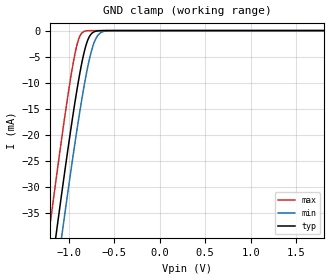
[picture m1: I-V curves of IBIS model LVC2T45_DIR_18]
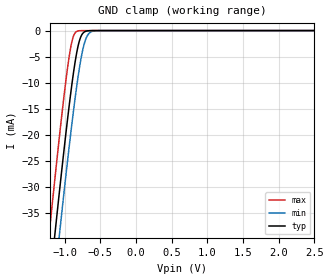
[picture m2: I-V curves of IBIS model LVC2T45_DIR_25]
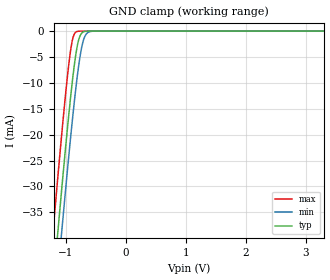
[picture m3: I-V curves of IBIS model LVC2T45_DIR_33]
| TEXAS INSTRUMENTS INCORPORATED
| Standard Linear and Logic Group
| IBIS Model of SN74LVC2T45
| 2-Bit Dual Supply Transceiver with Configurable Output Voltage
| This file contains package information for the following:
|  DSBGA 8-pin (YEP) package as [Component] LVC2T45_YEP
|  DSBGA 8-pin (YZP) package as [Component] LVC2T45_YZP
|  SOT 8-pin (DCT) package as [Component] LVC2T45_DCT
|  SOT 8-pin (DCU) package as [Component] LVC2T45_DCU
| This device can be powered at the following Vccs:
|  1.8 volt Vcc
|  2.5 volt Vcc
|  3.3 volt Vcc
|  5 volt Vcc
| This file provides unique models under the [Model Selector] for each Vcc.
| For operation at a specific Vcc, select the appropriate model after each
| [Model Selector] keyword.
[IBIS Ver]   3.2
[Comment char]  |_char
[File Name]   sn74lvc2t45.ibs
[File Rev]   1.2 | x_die
[Date]   April 30, 2004
[Source]   Data created from TI-SPICE simulations at TI-SLL.
[Notes]   The following is an IBIS list for the LVC2T45.
   Please contact sllibis@ti.com with questions and
   comments concerning SLL IBIS models.
   - FILE REV HISTORY
   - 1.1 Release IBIS file on 02/05/04
   - 1.2 YEP and YZP packages released 04/30/04
   - Due to the fact that the Device is 5-V Input/Output
   tolarent, the output model has some Non-Monotonic Warnings.
   - Power clamp data deleted as there is no power-clamp diode.
[Disclaimer] Property of Texas Instruments Incorporated.  Unauthorized
   reproduction and/or distribution is strictly prohibited.
   This product is protected under copyright law.
   Created  2003, (C) Copyright  2003, Texas Instruments
   Incorporated, All Rights Reserved
   UNLESS THERE IS A SIGNED, WRITTEN AGREEMENT TO THE
   CONTRARY, TEXAS INSTRUMENTS (TI) IS PROVIDING THE IBIS
   MODELS  AND WITHOUT ANY WARRANTY, EXPRESSED OR
   IMPLIED.  TI assumes no liability for:
   1) the accuracy of the IBIS models provided to your
   company;
   2) the proper functioning of these IBIS Models in your
   design or for any resulting applications; or
   3) infringement of patents, copyrights or intellectual
   property rights resulting from your use of these IBIS
   models.
   TI provides IBIS Models as a service to our customers.
   You and your company shall not distribute, sell or give
   these models to anyone else without prior written
   permission from TI.
   TI reserves the right to make changes to our products or
   to discontinue any semiconductor product or service
   without notice, and advises our customers to obtain the
   latest version of relevant information to verify, before
   placing orders, that the information being relied on is
   current.
   Please be aware that your receipt and use of the IBIS
   information provided shall serve as acceptance of these
   terms and conditions.  If you do not accept these terms,
   you should return or destroy the IBIS models and any
   other accompanying information immediately.
| Component LVC2T45_YEP 8-pin DSBGA
[Component]   LVC2T45_YEP
[Manufacturer]   Texas Instruments, Inc.
[Package]
|   typ   min   max
R_pkg   1.000e-03   1.000e-03   1.000e-03
L_pkg   2.450e-11   2.400e-11   2.500e-11
C_pkg   6.550e-14   6.400e-14   6.700e-14
[Pin]   signal_name   model_name   R_pin   L_pin   C_pin
1   VCCA   POWER   1.000e-03   2.500e-11   6.400e-14
2   A1   LVC2T45_IO_A   1.000e-03   2.400e-11   6.700e-14
3   A2   LVC2T45_IO_A   1.000e-03   2.400e-11   6.700e-14
4   GND   GND   1.000e-03   2.500e-11   6.400e-14
5   DIR   LVC2T45_DIR   1.000e-03   2.500e-11   6.400e-14
6   B2   LVC2T45_IO_B   1.000e-03   2.400e-11   6.700e-14
7   B1   LVC2T45_IO_B   1.000e-03   2.400e-11   6.700e-14
8   VCCB   POWER   1.000e-03   2.500e-11   6.400e-14
| Component LVC2T45_YZP 8-pin DSBGA
[Component]   LVC2T45_YZP
[Manufacturer]   Texas Instruments, Inc.
[Package]
|   typ   min   max
R_pkg   1.000e-03   1.000e-03   1.000e-03
L_pkg   2.450e-11   2.400e-11   2.500e-11
C_pkg   6.550e-14   6.400e-14   6.700e-14
[Pin]   signal_name   model_name   R_pin   L_pin   C_pin
1   VCCA   POWER   1.000e-03   2.500e-11   6.400e-14
2   A1   LVC2T45_IO_A   1.000e-03   2.400e-11   6.700e-14
3   A2   LVC2T45_IO_A   1.000e-03   2.400e-11   6.700e-14
4   GND   GND   1.000e-03   2.500e-11   6.400e-14
5   DIR   LVC2T45_DIR   1.000e-03   2.500e-11   6.400e-14
6   B2   LVC2T45_IO_B   1.000e-03   2.400e-11   6.700e-14
7   B1   LVC2T45_IO_B   1.000e-03   2.400e-11   6.700e-14
8   VCCB   POWER   1.000e-03   2.500e-11   6.400e-14
| Component LVC2T45_DCT 8-pin SOT
[Component]   LVC2T45_DCT
[Manufacturer]   Texas Instruments, Inc.
[Package]
|   typ   min   max
R_pkg   2.900e-02   2.800e-02   3.100e-02
L_pkg   1.796e-09   1.666e-09   1.924e-09
C_pkg   2.310e-13   2.210e-13   2.420e-13
[Pin]   signal_name   model_name   R_pin   L_pin   C_pin
1   VCCA   POWER   3.100e-02   1.894e-09   2.230e-13
2   A1   LVC2T45_IO_A   2.800e-02   1.697e-09   2.370e-13
3   A2   LVC2T45_IO_A   3.000e-02   1.722e-09   2.390e-13
4   GND   GND   3.000e-02   1.861e-09   2.210e-13
5   DIR   LVC2T45_DIR   2.800e-02   1.924e-09   2.280e-13
6   B2   LVC2T45_IO_B   2.900e-02   1.736e-09   2.420e-13
7   B1   LVC2T45_IO_B   2.800e-02   1.666e-09   2.360e-13
8   VCCB   POWER   3.000e-02   1.871e-09   2.220e-13
| Component LVC2T45_DCU 8-pin SOT
[Component]   LVC2T45_DCU
[Manufacturer]   Texas Instruments, Inc.
[Package]
|   typ   min   max
R_pkg   2.600e-02   2.300e-02   3.800e-02
L_pkg   1.394e-09   1.066e-09   2.046e-09
C_pkg   2.590e-13   2.150e-13   3.720e-13
[Pin]   signal_name   model_name   R_pin   L_pin   C_pin
1   VCCA   POWER   2.400e-02   1.520e-09   2.710e-13
2   A1   LVC2T45_IO_A   2.300e-02   1.112e-09   2.180e-13
3   A2   LVC2T45_IO_A   2.300e-02   1.070e-09   2.170e-13
4   GND   GND   2.700e-02   2.046e-09   3.720e-13
5   DIR   LVC2T45_DIR   2.700e-02   1.542e-09   2.730e-13
6   B2   LVC2T45_IO_B   2.300e-02   1.100e-09   2.240e-13
7   B1   LVC2T45_IO_B   2.300e-02   1.066e-09   2.150e-13
8   VCCB   POWER   3.800e-02   1.696e-09   2.800e-13
| Model LVC2T45_DIR
[Model Selector]   LVC2T45_DIR
LVC2T45_DIR_18   1.8 volt Vcc
LVC2T45_DIR_25   2.5 volt Vcc
LVC2T45_DIR_33   3.3 volt Vcc
LVC2T45_DIR_50   5 volt Vcc
| Model LVC2T45_IO_A
[Model Selector]   LVC2T45_IO_A
LVC2T45_IO_A_18   1.8 volt Vcc
LVC2T45_IO_A_25   2.5 volt Vcc
LVC2T45_IO_A_33   3.3 volt Vcc
LVC2T45_IO_A_50   5 volt Vcc
| Model LVC2T45_IO_B
[Model Selector]   LVC2T45_IO_B
LVC2T45_IO_B_18   1.8 volt Vcc
LVC2T45_IO_B_25   2.5 volt Vcc
LVC2T45_IO_B_33   3.3 volt Vcc
LVC2T45_IO_B_50   5 volt Vcc
| Models and submodels in the file (12): LVC2T45_DIR_18 (Input), LVC2T45_DIR_25 (Input), LVC2T45_DIR_33 (Input), LVC2T45_DIR_50 (Input), LVC2T45_IO_A_18 (I/O), LVC2T45_IO_A_25 (I/O), LVC2T45_IO_A_33 (I/O), LVC2T45_IO_A_50 (I/O), LVC2T45_IO_B_18 (I/O), LVC2T45_IO_B_25 (I/O), LVC2T45_IO_B_33 (I/O), LVC2T45_IO_B_50 (I/O)
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[Model]   LVC2T45_DIR_18
Model_type  Input
Vinl=0.5775
Vinh=1.2675
| variable   typ   min   max
C_comp   3.34pF   2.91pF   4.03pF
[Temperature Range]   40   100   -40
| Ambient temperature   25   85   -40
[Voltage range]   1.8   1.65   1.95
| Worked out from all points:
|   GND clamp passes 1 mA (typ) near -0.77 V on its own axis
[GND Clamp]
| LVC2T45_DIR_18
|   Voltage   I(typ)   I(min)   I(max)
-5.5V     -655.2mA   -662.2mA   -646.6mA
-1.215V   -49.6mA    -57.88mA   -38.96mA
-1.135V   -39.07mA   -47.36mA   -28.42mA
-1.075V   -31.35mA   -39.6mA    -20.75mA
-1.055V   -28.82mA   -37.05mA   -18.27mA
-955mV    -16.68mA   -24.66mA   -6.874mA
-885mV    -9.098mA   -16.55mA   -1.486mA
-825mV    -3.922mA   -10.26mA   -137.1uA
-780mV    -1.472mA   -6.227mA   -17.15uA
-715mV    -205.4uA   -2.128mA   -808.5nA
-650mV    -22.01uA   -443.9uA   -37.93nA
1.8V      3.326pA    6.142pA    3.026pA
[Model]   LVC2T45_DIR_25
Model_type  Input
Vinl=0.7
Vinh=1.7
| variable   typ   min   max
C_comp   3.24pF   2.69pF   4.07pF
[Temperature Range]   40   100   -40
| Ambient temperature   25   85   -40
[Voltage range]   2.5   2.3   2.7
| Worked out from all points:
|   GND clamp passes 1 mA (typ) near -0.77 V on its own axis
[GND Clamp]
| LVC2T45_DIR_25
|   Voltage   I(typ)   I(min)   I(max)
-5.5V     -655.2mA   -662.2mA   -646.6mA
-1.215V   -49.6mA    -57.88mA   -38.96mA
-1.14V    -39.72mA   -48.01mA   -29.07mA
-1.12V    -37.12mA   -45.41mA   -26.48mA
-1.08V    -31.98mA   -40.25mA   -21.38mA
-1.06V    -29.44mA   -37.69mA   -18.89mA
-960mV    -17.26mA   -25.26mA   -7.377mA
-890mV    -9.597mA   -17.1mA    -1.734mA
-785mV    -1.671mA   -6.635mA   -21.67uA
-720mV    -242.5uA   -2.354mA   -1.023uA
-650mV    -22.01uA   -443.9uA   -37.93nA
2.5V      4.713pA    7.577pA    4.389pA
[Model]   LVC2T45_DIR_33
Model_type  Input
Vinl=0.8
Vinh=2.0
| variable   typ   min   max
C_comp   3.15pF   2.57pF   4.08pF
[Temperature Range]   40   100   -40
| Ambient temperature   25   85   -40
[Voltage range]   3.3   3   3.6
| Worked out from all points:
|   GND clamp passes 1 mA (typ) near -0.77 V on its own axis
[GND Clamp]
| LVC2T45_DIR_33
|   Voltage   I(typ)   I(min)   I(max)
-5.5V     -655.2mA   -662.2mA   -646.6mA
-1.225V   -50.93mA   -59.21mA   -40.3mA
-1.145V   -40.37mA   -48.66mA   -29.72mA
-1.12V    -37.12mA   -45.41mA   -26.48mA
-1.08V    -31.98mA   -40.25mA   -21.38mA
-1.06V    -29.44mA   -37.69mA   -18.89mA
-965mV    -17.84mA   -25.87mA   -7.89mA
-885mV    -9.098mA   -16.55mA   -1.486mA
-780mV    -1.472mA   -6.227mA   -17.15uA
-715mV    -205.4uA   -2.128mA   -808.5nA
-640mV    -15.53uA   -338.1uA   -23.69nA
3.3V      6.304pA    9.258pA    5.93pA
